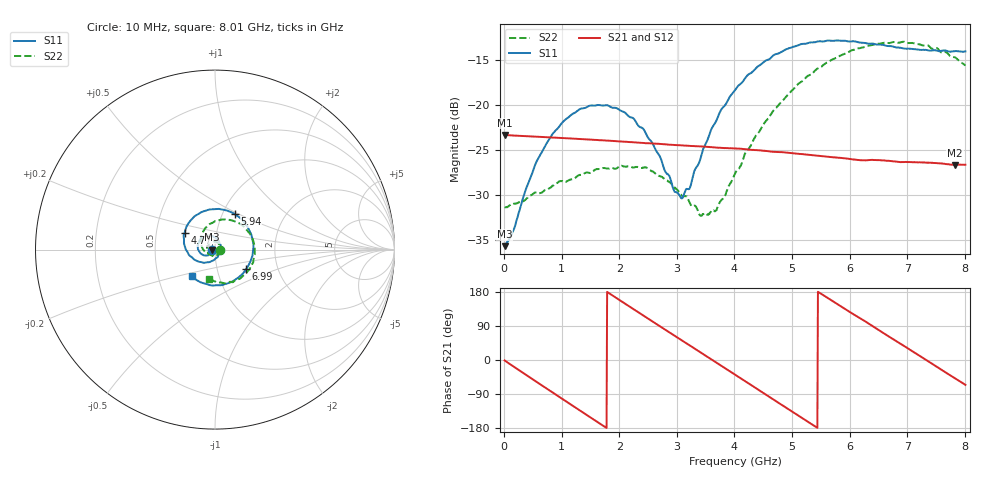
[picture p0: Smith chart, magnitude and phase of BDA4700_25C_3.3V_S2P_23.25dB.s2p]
!Agilent Technologies,E5071B,MY42404982,A.09.10
!Date: Mon Oct 20 18:12:49 2025
!Data & Calibration Information:
!Freq	S11:SOLT2(ON)	S21:SOLT2(ON)	S12:SOLT2(ON)	S22:SOLT2(ON)
# Hz S RI R 50
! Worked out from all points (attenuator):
!   801 points, 10 MHz to 8.01 GHz, reference 50 ohm
!   highest |S21| = -23.32 dB at 10 MHz (marker M1); lowest = -26.6 dB at 7.83 GHz (marker M2)
!   lowest |S11| = -35.7 dB at 10 MHz (marker M3), VSWR 1.03, Z = 48.4 - j0.106 ohm
!   |S11| at or under -10 dB: start of sweep to end of sweep
!   |S22| runs from -32.3 to -13.0 dB; largest |S21 - S12| = 0.00083
!   S11 on the Smith chart (normalised r, x): 10 MHz: 0.97, -0.00; 4.77 GHz: 0.70, +0.13; 5.94 GHz: 1.14, +0.48; 6.99 GHz: 1.38, -0.32; 8.01 GHz: 0.74, -0.23
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1e7  -0.0164 -0.00109  0.0682 -0.00149  0.0682 -0.0015  0.0271 -0.000767
1.5e8  -0.0175 -0.0094  0.0652 -0.0182  0.0652 -0.0182  0.0272 -0.00734
4e8  -0.0258 -0.0242  0.0506 -0.0441  0.0506 -0.0441  0.0214 -0.0217
7e8  -0.0479 -0.033  0.0213 -0.0628  0.0213 -0.0628  0.00608 -0.033
1.35e9  -0.0957 0.00511  -0.047 -0.0445  -0.0469 -0.0445  -0.0368 -0.018
2.08e9  -0.052 0.0755  -0.0547 0.0305  -0.0547 0.0305  -0.0299 0.0344
2.42e9  -0.00741 0.0732  -0.0282 0.0548  -0.0282 0.0547  -0.00454 0.0446
2.68e9  0.0203 0.0494  -0.00171 0.0609  -0.00184 0.0608  0.0137 0.0381
2.96e9  0.0313 0.0107  0.0261 0.054  0.026 0.0539  0.0267 0.0226
3.1e9  0.0287 -0.0105  0.0381 0.046  0.0378 0.0461  0.0292 0.0111
3.23e9  0.021 -0.0279  0.0468 0.0364  0.0469 0.0363  0.0283 0.00193
3.54e9  -0.0162 -0.0629  0.058 0.00757  0.0581 0.00751  0.0139 -0.0205
3.69e9  -0.0424 -0.0706  0.0576 -0.00724  0.0576 -0.00744  0.00123 -0.0261
4.01e9  -0.1041 -0.0611  0.0448 -0.0358  0.0449 -0.0357  -0.0319 -0.0265
4.77e9  -0.1697 0.0922  -0.0218 -0.0503  -0.0214 -0.0505  -0.0791 0.0616
5.35e9  -0.0664 0.2123  -0.052 -0.009  -0.0519 -0.0093  -0.0159 0.1484
5.94e9  0.1108 0.1976  -0.0342 0.0372  -0.0343 0.037  0.1184 0.1535
6.68e9  0.2117 -0.0123  0.0229 0.0433  0.0231 0.0432  0.2207 -0.00134
6.99e9  0.1735 -0.1095  0.0406 0.0261  0.0407 0.026  0.2046 -0.0847
7.45e9  0.0453 -0.1959  0.0467 -0.00977  0.0467 -0.00983  0.1113 -0.1717
7.83e9  -0.0807 -0.182  0.0311 -0.0346  0.031 -0.0347  0.0115 -0.1833
8.01e9  -0.1306 -0.149  0.0192 -0.0425  0.0193 -0.0424  -0.0324 -0.1623
